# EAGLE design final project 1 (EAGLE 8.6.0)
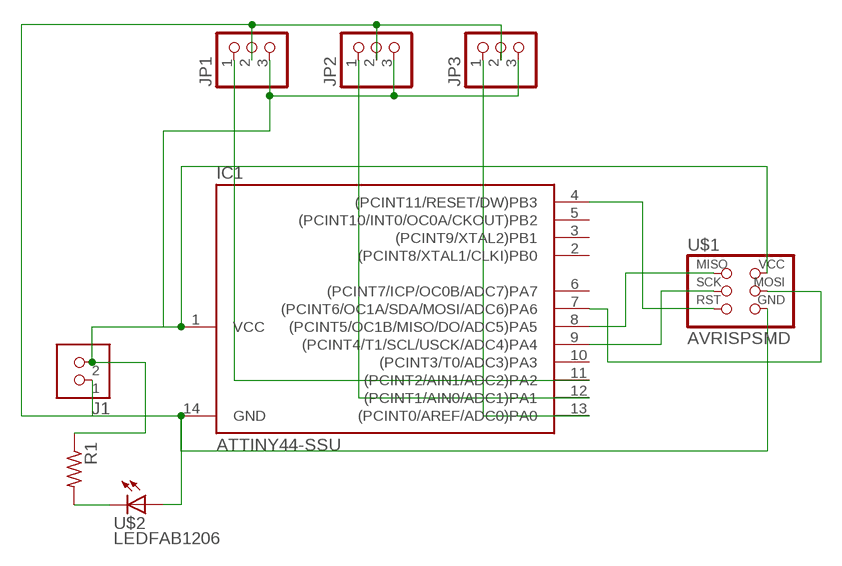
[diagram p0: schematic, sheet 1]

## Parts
IC1  ATTINY44-SSU  [SOIC14]
J1  TERM-1X02-FABLAB  [ED555DS-2DS]
JP1  PINHD-1X3  [1X03]
JP2  PINHD-1X3  [1X03]
JP3  PINHD-1X3  [1X03]
R1  RES-US1206FAB  [R1206FAB]
U$1  AVRISPSMD  [2X03SMD]
U$2  LEDFAB1206  [LED1206FAB]

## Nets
N$1: R1.2 U$2.2(C)
N$3: IC1.4((PCINT11/RESET/DW)PB3) U$1.5(RST)
N$4: IC1.9((PCINT4/T1/SCL/USCK/ADC4)PA4) U$1.3(SCK)
N$5: IC1.8((PCINT5/OC1B/MISO/DO/ADC5)PA5) U$1.1(MISO)
N$6: IC1.7((PCINT6/OC1A/SDA/MOSI/ADC6)PA6) U$1.4(MOSI)
N$7: IC1.14(GND) J1.1 JP1.2 JP2.2 JP3.2 U$1.6(GND) U$2.1(A)
N$8: IC1.13((PCINT0/AREF/ADC0)PA0) JP3.1
N$9: IC1.1(VCC) J1.2 JP1.3 JP2.3 JP3.3 R1.1 U$1.2(VCC)
N$10: IC1.12((PCINT1/AIN0/ADC1)PA1) JP2.1
N$11: IC1.11((PCINT2/AIN1/ADC2)PA2) JP1.1
Unconnected: IC1.2((PCINT8/XTAL1/CLKI)PB0) IC1.3((PCINT9/XTAL2)PB1) IC1.5((PCINT10/INT0/OC0A/CKOUT)PB2) IC1.6((PCINT7/ICP/OC0B/ADC7)PA7) IC1.10((PCINT3/T0/ADC3)PA3)

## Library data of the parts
IC1 = fab:ATTINY44
J1 = fab:TERM-1X02: 3.5mm terminal block, 2 positions ED555-2DS as found in the fablab inventory.
JP1-JP3 = pinhead:PINHD-1X3: PIN HEADER
R1 = fab:RES-US: Resistor (US Symbol)
U$1 = fab:AVRISP
U$2 = fab:LED: LED

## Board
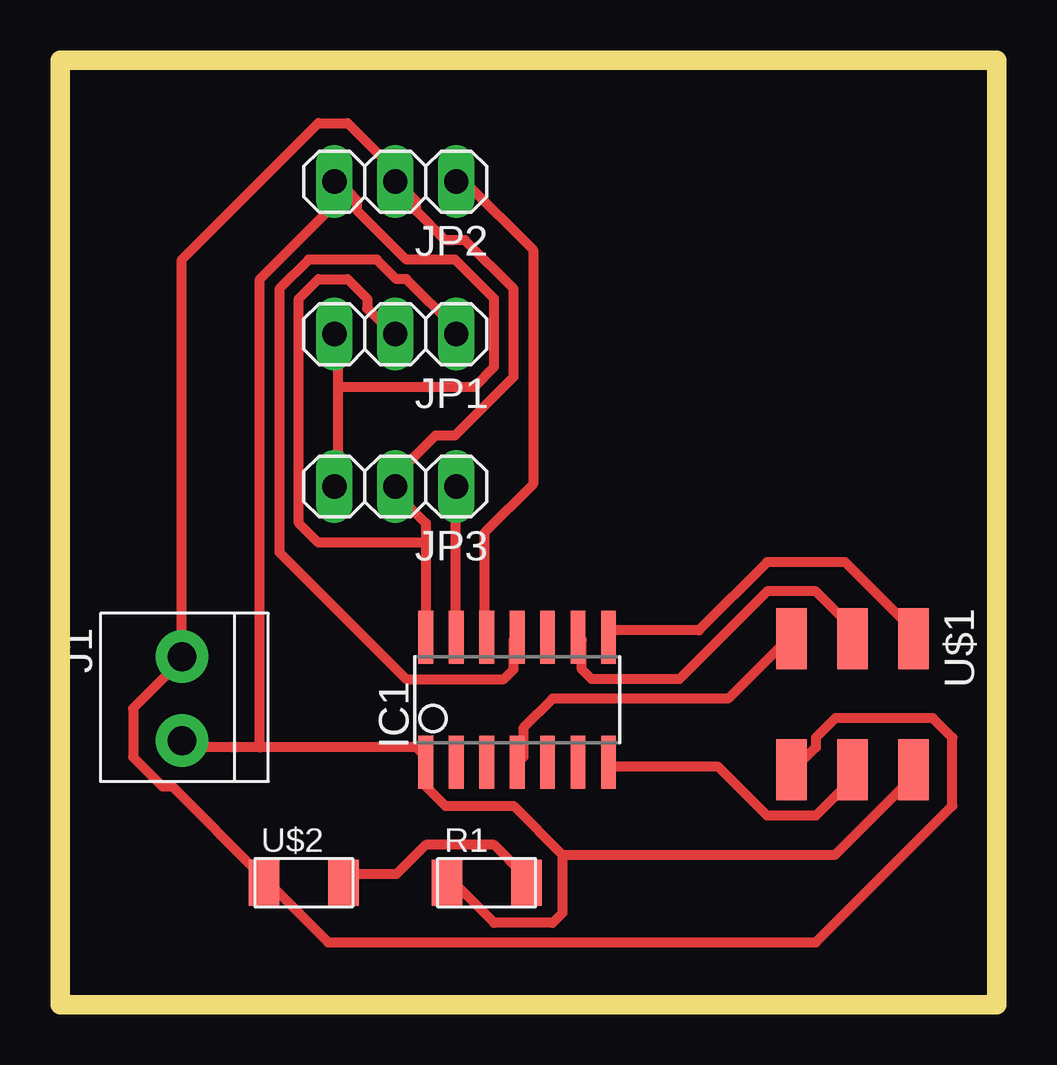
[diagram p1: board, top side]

Size 39.04 x 39.36 mm. Coordinates in mm from the lower left corner, seen from the top.
Outline: 0,0 39.04,0 39.04,39.36 0,39.36 0,0
Copper layers (1*16): Top 0.035mm / dielectric 1.5mm / Bottom 0.035mm
Design rules "default *": minimum track width 16mil, minimum drill 0.35mm, track to track 16mil, track to pad 16mil, pad to pad 16mil, via to via 16mil, smd to smd 16mil, copper to edge 40mil, drill to drill 16mil, minimum pad ring 10mil, minimum via ring 8mil, stop-mask expansion 4mil, vias tented up to drill 0mil, thermal gap 10mil

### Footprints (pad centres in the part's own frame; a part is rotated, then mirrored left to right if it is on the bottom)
SOIC14 = smd 0.61 x 2.21: 1 -3.81,-2.603; 2 -2.54,-2.603; 3 -1.27,-2.603; 4 0,-2.603; 5 1.27,-2.603; 6 2.54,-2.603; 7 3.81,-2.603; 8 3.81,2.603; 9 2.54,2.603; 10 1.27,2.603; 11 0,2.603; 12 -1.27,2.603; 13 -2.54,2.603; 14 -3.81,2.603
ED555DS-2DS = drill 1.2 pad 2.184: 1 1.8,0; 2 -1.7,0
1X03 = drill 1.016 long: 1 -2.54,0; 2 0,0; 3 2.54,0
R1206FAB = smd 1.27 x 1.905: 1 -1.651,0; 2 1.651,0
2X03SMD = smd 2.54 x 1.27: 1 -2.54,2.54; 2 2.92,2.54; 3 -2.54,0; 4 2.92,0; 5 -2.54,-2.54; 6 2.92,-2.54
LED1206FAB = smd 1.27 x 1.905: 1 -1.651,0; 2 1.651,0

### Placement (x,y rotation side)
IC1  19.05,12.7 0 top
J1  5.08,12.7 90 top
JP1  13.97,27.94 180 top
JP2  13.97,34.29 180 top
JP3  13.97,21.59 180 top
R1  17.78,5.08 0 top
U$1  33.02,12.7 270 top
U$2  10.16,5.08 0 top

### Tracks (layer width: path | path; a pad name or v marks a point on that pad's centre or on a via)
N$1
  Top 0.406: U$2.2 11.99,5.44 14.02,5.44 15.24,6.66 18.09,6.66 19.3,5.44 R1.2
N$3
  Top 0.406: IC1.4 19.3,10.31 19.3,11.53 20.52,12.75 27.84,12.75 30.28,15.19 U$1.5
N$4
  Top 0.406: IC1.9 21.74,15.19 21.74,13.97 22.15,13.56 25.81,13.56 29.46,17.22 31.5,17.22 33.12,15.6 U$1.3
N$5
  Top 0.406: IC1.8 22.96,15.6 26.62,15.6 29.46,18.44 32.72,18.44 35.56,15.6 U$1.1
N$6
  Top 0.406: IC1.7 22.96,9.91 27.43,9.91 29.46,7.87 31.5,7.87 33.12,9.5 U$1.4
N$7
  Top 0.406: 15.24,19.25 15.24,20.07 14.02,21.28 JP3.2 13.61,21.69 15.65,23.72 16.46,23.72 18.9,26.16 18.9,29.82 16.87,31.85 16.05,31.85 14.83,33.07 14.83,33.48 14.02,34.29 JP2.2 13.61,34.29 13.61,35.1 11.99,36.73 10.77,36.73 5.08,31.04 J1.1 5.08,14.38 3.05,12.34 3.05,10.31 4.27,9.09 4.67,9.09 8.33,5.44 U$2.1 8.74,5.03 11.18,2.59 31.5,2.59 37.19,8.28 37.19,11.12 36.37,11.94 32.31,11.94 31.5,11.12 31.5,10.72 30.68,9.91 U$1.6 | 15.24,19.25 IC1.14 | 15.24,19.25 10.77,19.25 9.96,20.07 9.96,29.41 10.77,30.23 11.99,30.23 12.8,29.41 12.8,29.01 13.61,28.19 JP1.2
N$8
  Top 0.406: IC1.13 16.46,15.6 16.46,21.28 JP3.1
N$9
  Top 0.406: 11.58,25.76 11.58,27.79 JP1.3 | 11.58,25.76 11.58,21.69 JP3.3 | 11.99,33.88 12.39,33.48 12.39,33.07 14.43,31.04 16.46,31.04 18.09,29.41 18.09,26.57 17.27,25.76 11.58,25.76 | 11.99,33.88 11.58,34.29 JP2.3 11.99,33.88 | 20.93,6.25 20.93,3.81 20.52,3.4 18.09,3.4 16.46,5.03 R1.1 | 20.93,6.25 18.9,8.28 16.05,8.28 15.24,9.09 IC1.1 15.24,10.31 14.83,10.72 8.33,10.72 | 20.93,6.25 32.31,6.25 35.56,9.5 U$1.2 | 8.33,10.72 5.08,10.72 J1.2 | 11.99,33.88 8.33,30.23 8.33,10.72
N$10
  Top 0.406: IC1.12 17.68,15.6 17.68,19.66 19.71,21.69 19.71,31.45 16.87,34.29 JP2.1
N$11
  Top 0.406: IC1.11 18.9,15.19 18.9,13.97 18.49,13.56 14.43,13.56 9.14,18.85 9.14,29.82 10.36,31.04 13.21,31.04 14.02,30.23 14.43,30.23 16.46,28.19 JP1.1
